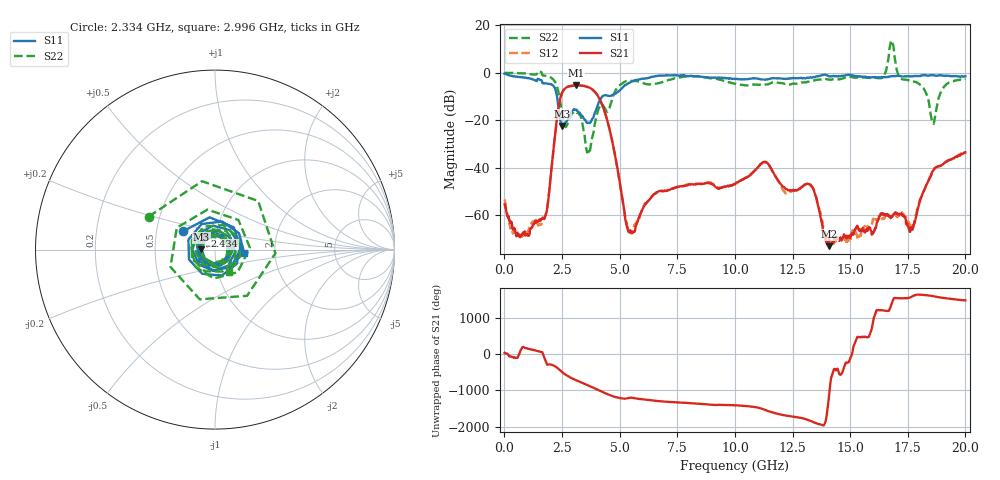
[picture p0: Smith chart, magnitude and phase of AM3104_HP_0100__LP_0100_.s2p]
!Created with skrf (http://scikit-rf.org).
# Hz S RI R 50.0
!freq ReS11 ImS11 ReS21 ImS21 ReS12 ImS12 ReS22 ImS22
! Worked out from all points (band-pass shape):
!   1601 points, 10 MHz to 20 GHz, reference 50 ohm
!   highest |S21| = -5.25 dB at 3.108 GHz (marker M1); lowest = -73.1 dB at 14.1 GHz (marker M2)
!   |S21| within 3 dB of the highest: 2.511 GHz to 3.945 GHz (1.434 GHz wide, 44.4 % of centre)
!   lowest |S11| = -22.5 dB at 2.521 GHz (marker M3), VSWR 1.16, Z = 43 + j0.0722 ohm
!   |S11| at or under -10 dB: 2.285 GHz to 4.243 GHz (1.958 GHz wide, 60 % of centre)
!   |S22| runs from -34.2 to 13.6 dB; largest |S21 - S12| = 0.03
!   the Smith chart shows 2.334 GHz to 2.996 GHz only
!   S11 on the Smith chart (normalised r, x): 2.334 GHz: 0.68, +0.15; 2.434 GHz: 0.89, +0.14; 2.996 GHz: 1.39, -0.06
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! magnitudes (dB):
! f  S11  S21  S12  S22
! 10 MHz  -0.4  -55.4  -53.4  0.0
! 697.2 MHz  -1.9  -68.8  -68.8  -0.2
! 1.659 GHz  -4.4  -61.0  -62.6  -1.1
! 2.334 GHz  -13.7  -15.5  -15.5  -7.7
! 2.434 GHz  -20.5  -10.5  -10.5  -12.9
! 2.521 GHz  -22.5  -8.1  -8.1  -18.3
! 2.996 GHz  -15.7  -5.3  -5.4  -16.7
! 3.108 GHz  -15.6  -5.3  -5.2  -16.6
! 3.346 GHz  -17.9  -5.4  -5.4  -19.3
! 3.646 GHz  -21.1  -6.1  -6.2  -33.2
! 4.358 GHz  -9.4  -16.7  -16.7  -15.0
! 5.407 GHz  -4.3  -67.2  -66.8  -3.4
! 6.682 GHz  -1.2  -50.0  -50.4  -4.4
! 10.01 GHz  -2.7  -47.0  -46.9  -4.6
! 11.3 GHz  -2.9  -37.5  -37.8  -4.9
! 13.34 GHz  -2.1  -48.1  -47.9  -3.5
! 14.1 GHz  -1.5  -73.1  -71.0  -2.9
! 16.35 GHz  -1.9  -59.2  -61.7  -2.3
! 16.68 GHz  -1.6  -60.6  -59.9  7.2
! 17.66 GHz  -1.5  -65.7  -65.2  -3.7
! 18.59 GHz  -1.0  -41.4  -41.8  -21.1
! 20 GHz  -1.4  -33.6  -33.3  -2.5
